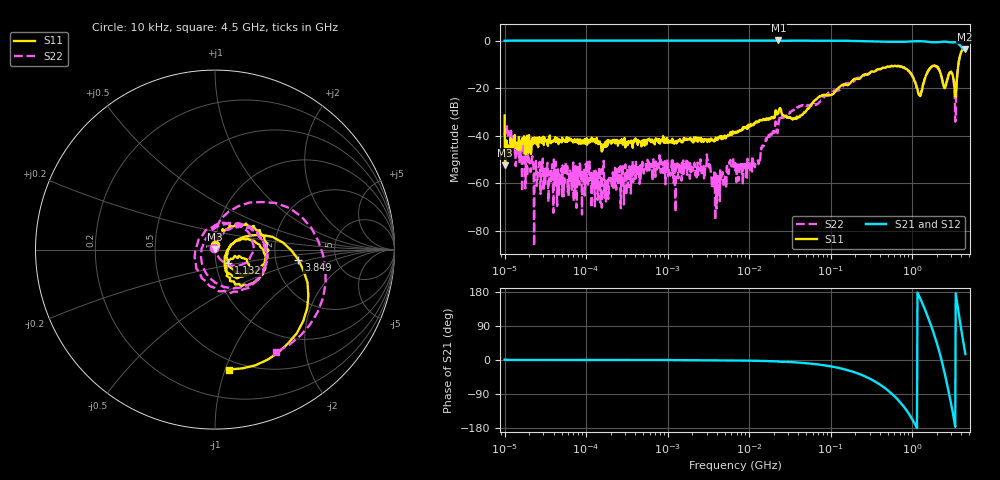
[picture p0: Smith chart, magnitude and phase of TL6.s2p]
!Siglent Technologies,SNA5004A,SNA5XCED5R0097,V1.0.0.2.10.R9
!Date: 2024-11-24 16:45:57
!Data & Calibration Information:
!Freq	S11:F2(ON)	S21:F2(ON)	S12:F2(ON)	S22:F2(ON)
# Hz S DB R 50
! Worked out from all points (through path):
!   1001 points, 10 kHz to 4.5 GHz, reference 50 ohm
!   highest |S21| = 0.10 dB at 22.8 MHz (marker M1); lowest = -3.7 dB at 4.442 GHz (marker M2)
!   group delay of S21, straight-line fit = 440 ps
!   lowest |S11| = -52.4 dB at 10.13 kHz (marker M3), VSWR 1.00, Z = 49.9 + j0.211 ohm
!   |S11| at or under -10 dB: start of sweep to 3.693 GHz
!   |S22| runs from -86.3 to -3.4 dB; largest |S21 - S12| = 0.02
!   S11 on the Smith chart (normalised r, x): 10 kHz: 1.00, +0.05; 1.132 GHz: 1.14, -0.17; 3.849 GHz: 2.70, -0.40; 4.5 GHz: 0.42, -1.03
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10000  -31.44 89.3  -0.02 0.9  -0.05 0.9  -39.82 121.9
10131.02  -52.37 118.5  -0.02 0.3  -0.07 0.2  -37.87 121.0
24233.63  -43.09 22.2  0.05 0.2  -0.01 0.1  -50.51 98.3
87919.76  -43.22 11.1  0.06 0.0  0.00 -0.1  -54.64 -46.7
772988.4  -42.77 20.7  0.06 -0.1  0.00 -0.3  -51.15 -39.6
3112194  -41.91 26.2  0.07 -0.6  0.01 -0.8  -49.86 -36.8
4090573  -41.51 45.7  0.05 -0.7  -0.01 -0.9  -56.94 -62.9
6708204  -38.51 70.0  0.04 -1.1  -0.03 -1.3  -51.40 159.2
1.253027e7  -34.27 83.3  0.05 -2.2  -0.03 -2.3  -50.99 99.8
2.280385e7  -30.53 106.0  0.10 -4.0  0.02 -4.0  -36.31 86.2
5.897837e7  -26.60 69.7  -0.00 -10.0  -0.07 -10.0  -26.91 86.4
2.313556e8  -15.71 52.2  -0.17 -38.0  -0.24 -37.8  -15.49 50.7
5.185364e8  -11.01 13.3  -0.47 -82.3  -0.53 -82.0  -10.88 2.0
8.072136e8  -11.36 -24.2  -0.46 -125.8  -0.51 -125.5  -11.44 -48.0
1.132327e9  -19.58 -46.0  -0.20 -177.1  -0.25 -176.8  -19.05 -128.5
1.673279e9  -11.35 -0.4  -0.59 95.9  -0.65 96.2  -11.52 12.8
2.257315e9  -14.22 -64.4  -0.50 5.9  -0.57 6.4  -14.70 -105.5
2.890702e9  -13.33 -28.0  -0.67 -97.3  -0.72 -96.5  -13.37 20.1
3.379417e9  -23.38 -36.6  -0.66 -176.4  -0.74 -175.7  -34.01 -74.7
3.849231e9  -6.59 -7.1  -1.85 103.4  -1.92 104.1  -6.46 29.1
4.441803e9  -3.36 -76.8  -3.67 22.9  -3.74 24.0  -3.44 -52.0
4.5e9  -3.44 -83.1  -3.62 15.5  -3.67 16.8  -3.53 -59.2
